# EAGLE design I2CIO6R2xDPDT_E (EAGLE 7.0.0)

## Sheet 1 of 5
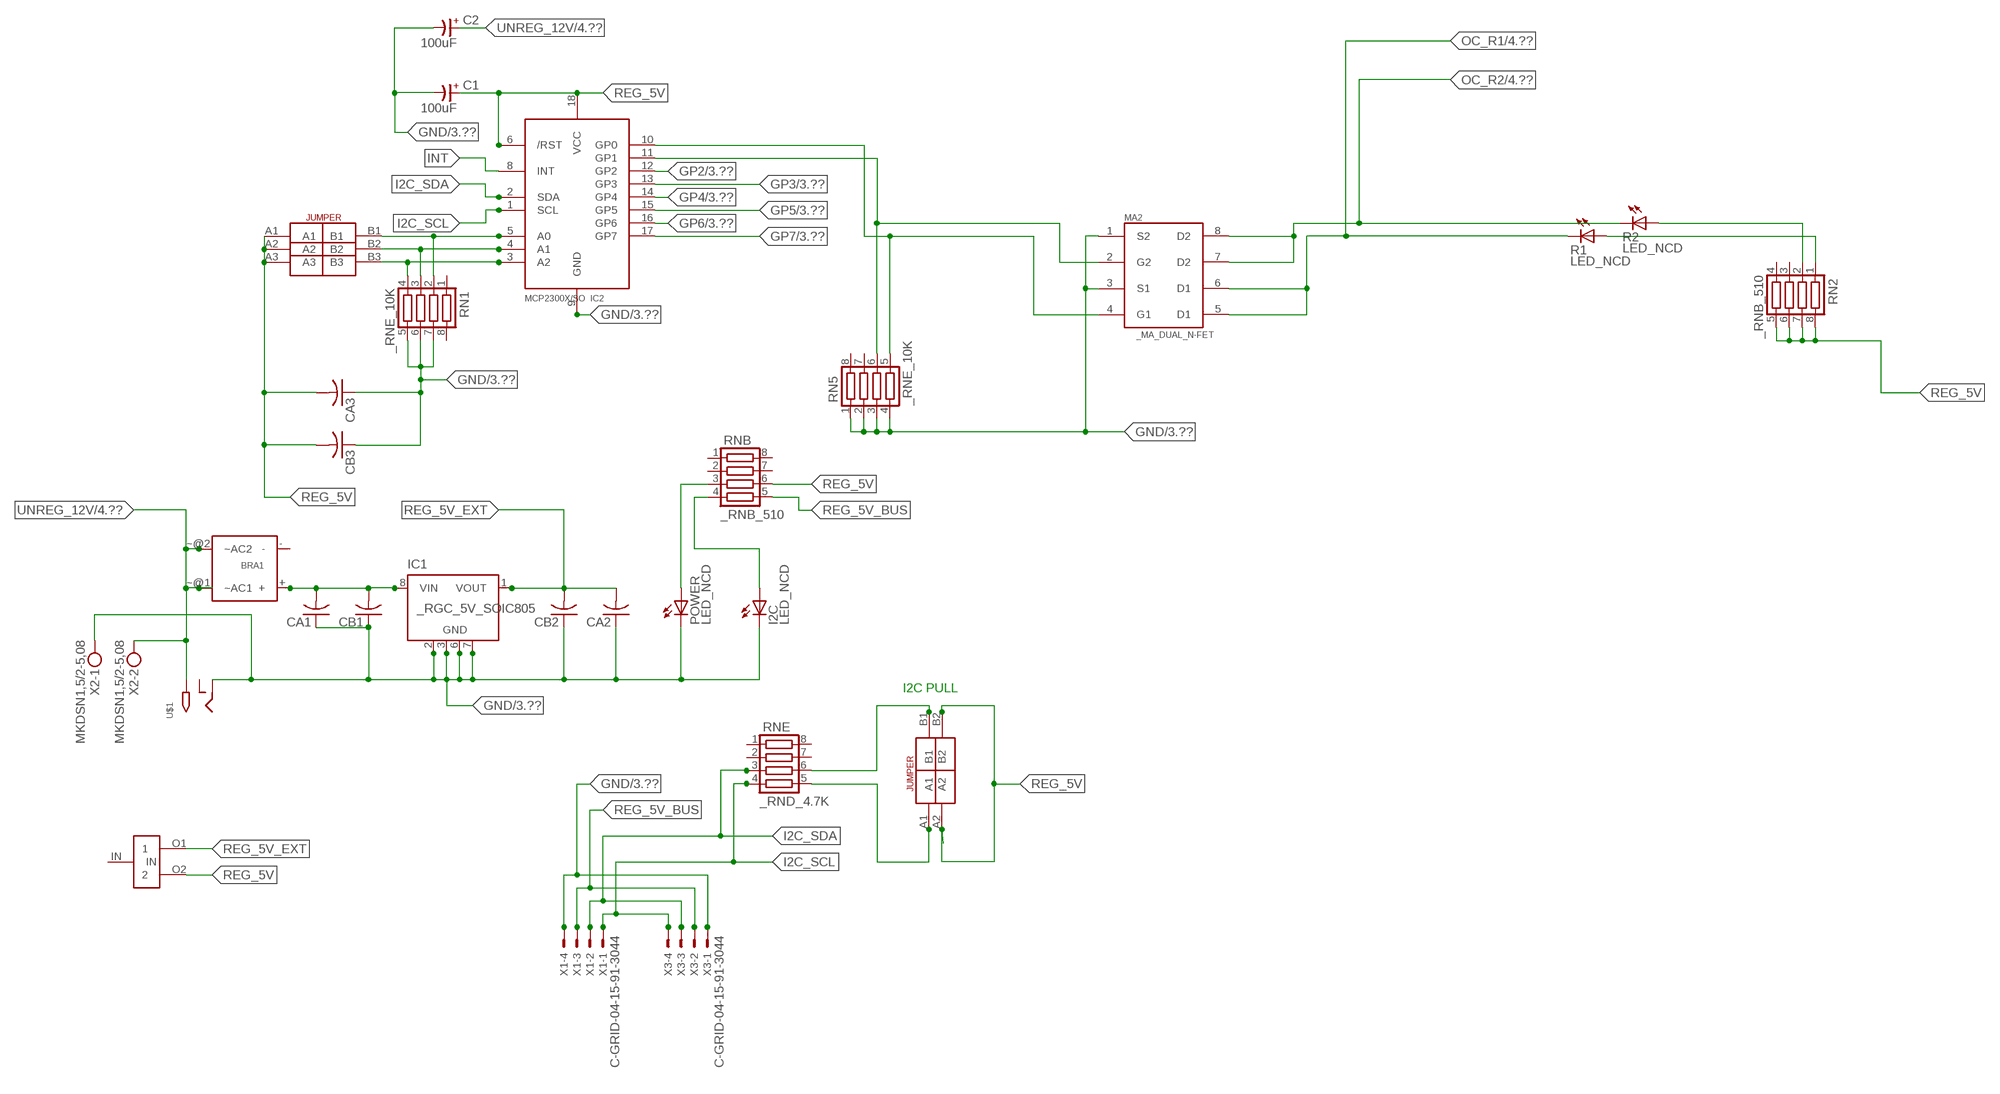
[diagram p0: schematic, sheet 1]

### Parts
BRA1  MB2S_  [MB2S]
C1  100uF  CP-E-025X060  [E-025X060]
C2  100uF  CP-E-025X060  [E-025X060]
CA1  CC1206KRX7R9BB104C1206K  [CC1206KRX7R9BB104]
CA2  CC1206KRX7R9BB104C1206K  [CC1206KRX7R9BB104]
CA3  CC1206KRX7R9BB104C1206K  [CC1206KRX7R9BB104]
CB1  TMK316F106ZL-TC1206K  [TMK316F106ZL-T]
CB2  TMK316F106ZL-TC1206K  [TMK316F106ZL-T]
CB3  TMK316F106ZL-TC1206K  [TMK316F106ZL-T]
I2C  LED_NCD  [CHIPLED_0603]
IC1  _RGC_5V_SOIC805  [_RGC_5V_SOIC8]
IC2  MCP2300X/SO  [SO18W]
MA2  _MA_DUAL_N-FET  [_MA_DUAL_N-FET]
POWER  LED_NCD  [CHIPLED_0603]
R1  LED_NCD  [CHIPLED_0603]
R2  LED_NCD  [CHIPLED_0603]
RN1  _RNE_10K  [RNE]
RN2  _RNB_510  [RNB]
RN5  _RNE_10K  [RNE]
RNB  _RNB_510  [RNB]
RNE  _RND_4.7K  [RND]
U$1  2.1MMJACK  [PJ-102A]
U$3  JUMPER_2X2  [JUMPER_2X2]
U$5  LINK_2  [LINK_2]
U$18  JUMPER_3X2  [JUMPER_3X2]
X1  C-GRID-04-15-91-3044  [15-91-04]
X2  MKDSN1,5/2-5,08  [MKDSN1,5/2-5,08]
X3  C-GRID-04-15-91-3044  [15-91-04]

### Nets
GND: C1.- C2.- CA1.1 CA2.1 CA3.1 CB1.1 CB2.1 CB3.1 I2C.C IC1.2(GND) IC1.3(GND) IC1.6(GND) IC1.7(GND) IC2.9(GND) MA2.1(S2) MA2.3(S1) POWER.C RN1.5 RN1.6 RN1.7 RN5.1 RN5.2 RN5.3 RN5.4 U$1.RING X1.4 X2.1 X3.1 ; also sheet 3
GP2: IC2.12(GP2) ; also sheet 3
GP3: IC2.13(GP3) ; also sheet 3
GP4: IC2.14(GP4) ; also sheet 3
GP5: IC2.15(GP5) ; also sheet 3
GP6: IC2.16(GP6) ; also sheet 3
GP7: IC2.17(GP7) ; also sheet 3
I2C_SCL: IC2.1(SCL) RNE.4 X1.1 X3.4
I2C_SDA: IC2.2(SDA) RNE.3 X1.2 X3.3
INT: IC2.8(INT)
N$1: BRA1.+ CA1.2 CB1.2 IC1.8(VIN)
N$2: POWER.A RNB.3
N$3: I2C.A RNB.4
N$4: RNE.5 U$3.A1
N$5: RNE.6 U$3.B1
N$6: IC2.5(A0) RN1.2 U$18.B1
N$7: IC2.4(A1) RN1.3 U$18.B2
N$8: IC2.3(A2) RN1.4 U$18.B3
N$22: IC2.11(GP1) MA2.2(G2) RN5.6
N$23: IC2.10(GP0) MA2.4(G1) RN5.5
N$31: R2.A RN2.2
N$32: R1.A RN2.1
OC_R1: MA2.5(D1) MA2.6(D1) R1.C ; also sheet 4
OC_R2: MA2.7(D2) MA2.8(D2) R2.C ; also sheet 4
REG_5V: C1.+ CA3.2 CB3.2 IC2.6(/RST) IC2.18(VCC) RN2.5 RN2.6 RN2.7 RN2.8 RNB.6 U$3.A2 U$3.B2 U$5.O2 U$18.A1 U$18.A2 U$18.A3
REG_5V_BUS: RNB.5 X1.3 X3.2
REG_5V_EXT: CA2.2 CB2.2 IC1.1(VOUT) U$5.O1
UNREG_12V: BRA1.~@1(~AC1) BRA1.~@2(~AC2) C2.+ U$1.TIP X2.2 ; also sheet 4
Unconnected: BRA1.- IC1.4(NC) IC1.5(NC) RN1.1 RN1.8 RN2.3 RN2.4 RN5.7 RN5.8 RNB.1 RNB.2 RNB.7 RNB.8 RNE.1 RNE.2 RNE.7 RNE.8 U$1.RING_SW U$5.IN

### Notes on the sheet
- I2C PULL

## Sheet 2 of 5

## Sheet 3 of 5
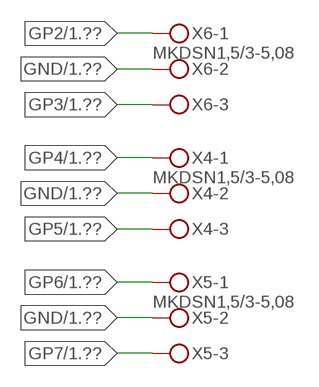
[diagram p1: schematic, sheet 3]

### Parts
X4  MKDSN1,5/3-5,08  [MKDSN1,5/3-5,08]
X5  MKDSN1,5/3-5,08  [MKDSN1,5/3-5,08]
X6  MKDSN1,5/3-5,08  [MKDSN1,5/3-5,08]

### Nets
GND: X4.2 X5.2 X6.2 ; also sheet 1
GP2: X6.1 ; also sheet 1
GP3: X6.3 ; also sheet 1
GP4: X4.1 ; also sheet 1
GP5: X4.3 ; also sheet 1
GP6: X5.1 ; also sheet 1
GP7: X5.3 ; also sheet 1

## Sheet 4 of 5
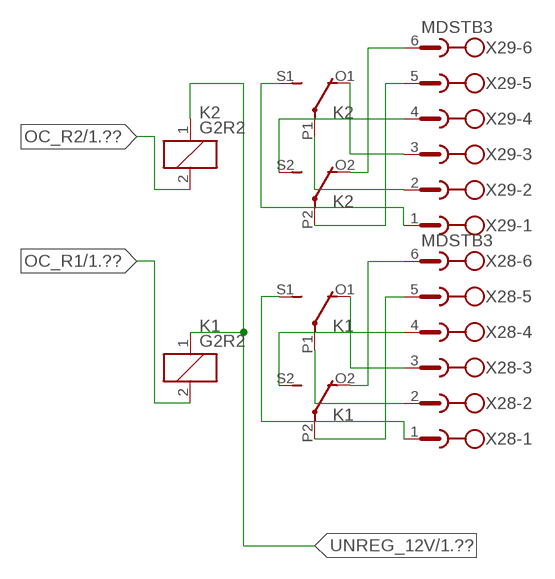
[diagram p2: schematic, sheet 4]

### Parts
K1  G2R2  [G2R2]
K2  G2R2  [G2R2]
X28  MDSTB3  [MDSTB3]
X29  MDSTB3  [MDSTB3]

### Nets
N$203: K1.P2(3:COM) X28.5
N$204: K1.O2(3:NC) X28.6
N$205: K1.S2(3:NO) X28.4
N$206: K1.P1(2:COM) X28.2
N$207: K1.O1(2:NC) X28.3
N$208: K1.S1(2:NO) X28.1
N$209: K2.P2(3:COM) X29.5
N$210: K2.O2(3:NC) X29.6
N$211: K2.S2(3:NO) X29.4
N$212: K2.S1(2:NO) X29.1
N$213: K2.P1(2:COM) X29.2
N$214: K2.O1(2:NC) X29.3
OC_R1: K1.2(1:C2) ; also sheet 1
OC_R2: K2.2(1:C2) ; also sheet 1
UNREG_12V: K1.1(1:C1) K2.1(1:C1) ; also sheet 1

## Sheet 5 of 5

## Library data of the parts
BRA1 = NCD_ULTIMATE_LIBRARY:MB2S: Bridge Rectifier BRA MB2S 200V 500ma Digikey MB2S-TPMSTR-ND/MB2S-TP
C1 C2 = NCD_ULTIMATE_LIBRARY:CP-: Capacitors All Kinds POLARIZED CAP
CA1-CA3 = NCD_ULTIMATE_LIBRARY:CC1206KRX7R9BB104: Capacitor CA .1uF 50V SMT C1206K CC1206KRX7R9BB104
CB1-CB3 = NCD_ULTIMATE_LIBRARY:TMK316F106ZL-T: Capacitor CB 10uF SMT 1206 TMK316F106ZL-T
I2C POWER = NCD_ULTIMATE_bhaskar:LED_NCD
IC1 = NCD_ULTIMATE_LIBRARY:_RGC_5V_SOIC8: Regulator Linear 5V Chip Positive VOLTAGE REGULATOR Digikey 497-7267-2-ND/L78L05CD13TR
IC2 = NCD_ULTIMATE_LIBRARY:MCP2300X: Semiconductor Port Expander I/O 8-Bit I2C MCP23008 Inexpensive i2c i/o expander - 8 general purpose i/o pins with optional pullups
K1 K2 = NCD_ULTIMATE_LIBRARY:G2R2: RELAY 2 x switch, Omron
MA2 = NCD_ULTIMATE_LIBRARY:_MA_DUAL_N-FET: FET Dual N-Channel 8-SOIC NMOSFET Digikey 785-1064-2-ND/AO4842
R1 R2 = NCD_ULTIMATE_LIBRARY:LED_NCD: LED Digikey 754-1132-2-ND/APT2012SRCPRV
RN1 RN5 = NCD_ULTIMATE_LIBRARY:_RNE_10K: Resistor Array RNE SMT 10K x 4 Single Resistor Source: http://www.ctscorp.com/components/Datasheets/CTSChipArrayDs.pdf Digikey 742C083103JPTR-ND/742C083103JP; OC_FARNELL: unknown; OC_NEWARK: unknown
RN2 RNB = NCD_ULTIMATE_LIBRARY:_RNB_510: Resistor Array RNB SMT 510 x 4 Single Resistor Source: http://www.ctscorp.com/components/Datasheets/CTSChipArrayDs.pdf Digikey 742C083511JPTR-ND/ 742C083511JP; OC_FARNELL: unknown; OC_NEWARK: unknown
RNE = NCD_ULTIMATE_LIBRARY:_RND_4.7K: Resistor Array RND SMT 4.7K x 4 Single Resistor Source: http://www.ctscorp.com/components/Datasheets/CTSChipArrayDs.pdf Digikey 742C083472JPTR-ND/742C083472JP; OC_FARNELL: unknown; OC_NEWARK: unknown
U$1 = NCD_ULTIMATE_CONNECTORS:2.1MMJACK: 2.1mm x 5.5mm DC jack with internal switch. Digikey part #PJ-102A, 4UCON part #05537 By microbuilder.eu
U$3 = NCD_ULTIMATE_CONNECTORS:JUMPER_2X2
U$5 = NCD_ULTIMATE_LIBRARY:LINK_2: PAD_top
U$18 = NCD_ULTIMATE_CONNECTORS:JUMPER_3X2
X1 X3 = NCD_ULTIMATE_CONNECTORS:C-GRID-04: CONNECTOR 4-Pos I2C wire to board 2.54 mm (0.100") pitch header Digikey WM1342-ND/0015912045; OC_FARNELL: unknown; OC_NEWARK: unknown
X2 = NCD_ULTIMATE_CONNECTORS:MKDSN1,5/2-5,08: MKDSN 1,5/ 2-5,08 Printklemme
X4-X6 = NCD_ULTIMATE_CONNECTORS:MKDSN1,5/3-5,08: MKDSN 1,5/ 3-5,08 Printklemme Nennstrom: 13,5 A Nennspannung: 250 V Rastermaß: 5,08 mm Polzahl: 3 Anschlussart: Schraubanschluss Montage: Löten Anschlussrichtung Leiter/Platine: 0 ° Artikelnummer: 1729131 Source: http://eshop.phoenixcontact.com .. 1729131.pdf
X28 X29 = NCD_ULTIMATE_LIBRARY:MDSTB3: PHOENIX

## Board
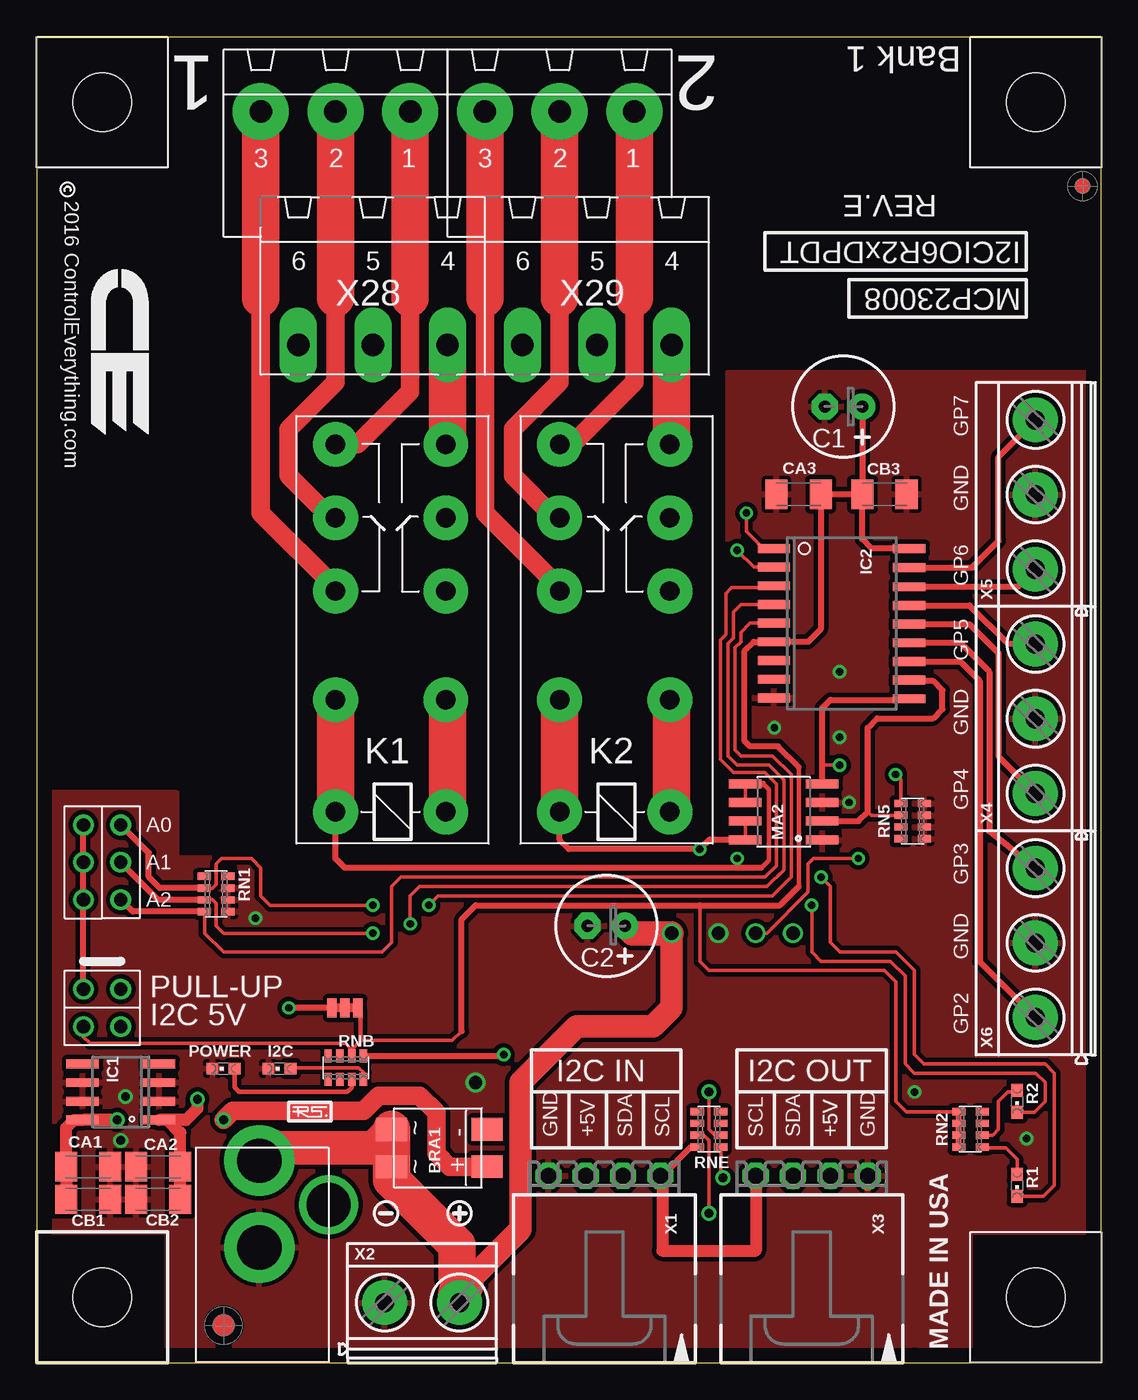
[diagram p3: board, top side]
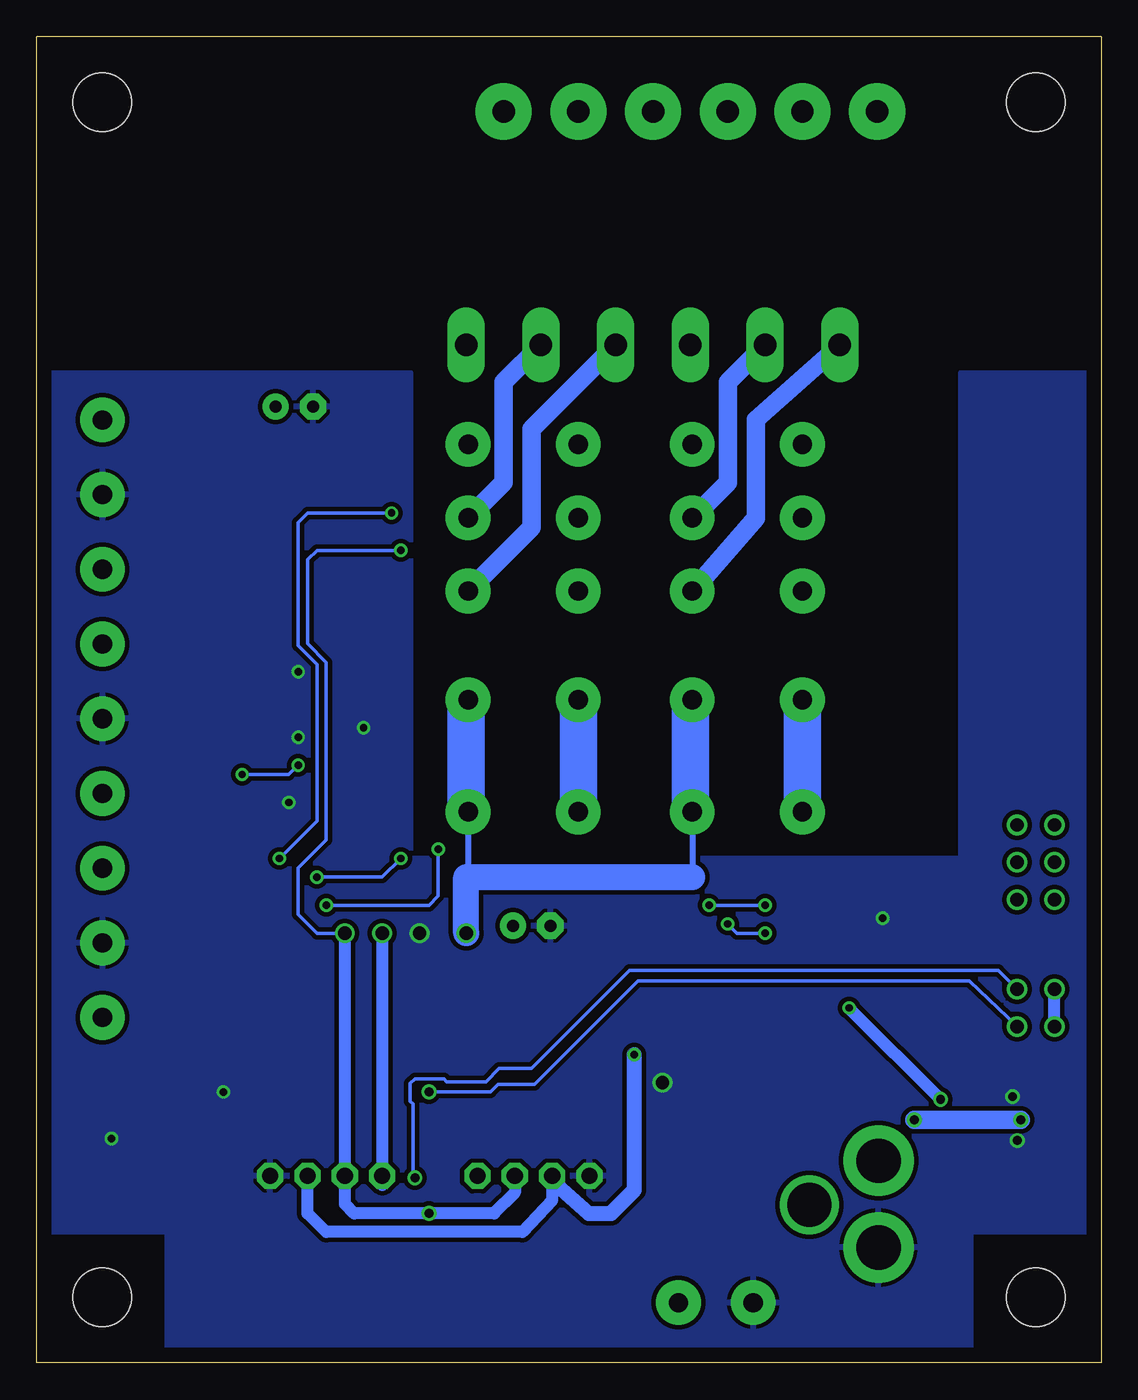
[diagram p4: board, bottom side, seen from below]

Size 72.39 x 90.17 mm. Coordinates in mm from the lower left corner, seen from the top.
Outline: 59.69,0 0,0 0,76.2 0,90.17 72.39,90.17 72.39,0 59.69,0
Outline: 59.69,0 61.58,0
Copper layers (1*16): Top 0.035mm / dielectric 1.5mm / Bottom 0.035mm
Design rules "default": minimum track width 10mil, minimum drill 24mil, track to track 8mil, track to pad 8mil, pad to pad 8mil, via to via 8mil, smd to smd 8mil, copper to edge 40mil, drill to drill 8mil, minimum pad ring 10mil, minimum via ring 8mil, stop-mask expansion 4mil, vias tented up to drill 0mil, thermal gap 10mil
Holes 3.96 mm at 4.45,4.45

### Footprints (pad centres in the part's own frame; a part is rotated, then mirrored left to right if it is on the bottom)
MB2S = smd 1.55 x 2.1: + 0,-6.5; - 2.54,-6.5; ~@1 0,0; ~@2 2.54,0
E-025X060 = drill 0.813 pad 1.778: + -1.27,0 | drill 0.813 pad 1.778 octagon: - 1.27,0
CC1206KRX7R9BB104 = smd 1.5 x 2: 1 -1.5,0; 2 1.5,0
TMK316F106ZL-T = smd 1.5 x 2: 1 -1.5,0; 2 1.5,0
CHIPLED_0603 = smd 0.8 x 0.8: A 0,-0.75; C 0,0.75
_RGC_5V_SOIC8 = smd 0.6 x 2.2: 1 -1.905,-2.6; 2 -0.635,-2.6; 3 0.635,-2.6; 4 1.905,-2.6; 5 1.905,2.6; 6 0.635,2.6; 7 -0.635,2.6; 8 -1.905,2.6
SO18W = smd 0.6 x 2.2: 1 -4.445,-4.6; 2 -3.175,-4.6; 3 -1.905,-4.6; 4 -0.635,-4.6; 5 0.635,-4.6; 6 1.905,-4.6; 7 3.175,-4.6; 8 4.445,-4.6; 9 5.715,-4.6; 10 5.775,4.6; 11 4.505,4.6; 12 3.235,4.6; 13 1.965,4.6; 14 0.695,4.6; 15 -0.575,4.6; 16 -1.845,4.6; 17 -3.145,4.6; 18 -4.445,4.6
G2R2 = drill 1.321 pad 3.048: 1 -2.54,-3.683; 2 -2.54,3.81; 3 5.08,-3.683; 4 5.08,3.81; O1 12.471,3.81; O2 12.471,-3.683; P1 17.45,3.81; P2 17.45,-3.683; S1 22.454,3.81; S2 22.454,-3.683
_MA_DUAL_N-FET = smd 0.61 x 2.21: 1 -1.905,-2.616; 2 -0.635,-2.616; 3 0.635,-2.616; 4 1.905,-2.616; 5 1.905,2.616; 6 0.635,2.616; 7 -0.635,2.616; 8 -1.905,2.616
CHIPLED_0603' = smd 0.8 x 0.876: A 0,-0.75; C 0,0.75
RNE = smd 0.5 x 0.9: 1 -1.2,-0.8; 2 -0.4,-0.8; 3 0.4,-0.8; 4 1.2,-0.8; 5 1.2,0.8; 6 0.4,0.8; 7 -0.4,0.8; 8 -1.2,0.8
RNB = smd 0.5 x 0.9: 1 -1.2,-0.8; 2 -0.4,-0.8; 3 0.4,-0.8; 4 1.2,-0.8; 5 1.2,0.8; 6 0.4,0.8; 7 -0.4,0.8; 8 -1.2,0.8
RND = smd 0.5 x 0.9: 1 -1.2,-0.8; 2 -0.4,-0.8; 3 0.4,-0.8; 4 1.2,-0.8; 5 1.2,0.8; 6 0.4,0.8; 7 -0.4,0.8; 8 -1.2,0.8
PJ-102A = drill 3 pad 4.8: RING 0.1,-3.39; TIP 0.1,-9.29 | drill 3 pad 3.251: RING_SW -4.6,-6.29
JUMPER_2X2 = drill 0.9: A1 0,2.54; A2 0,0; B1 2.54,2.54; B2 2.54,0
PCB_MOUNTING_HOLE = hole 3.962: 4.445,4.445
LINK_2 = smd 1.27 x 0.635: IN 0,0; O1 0,0.889; O2 0,-0.889
JUMPER_3X2 = drill 0.9: A1 0,5.08; A2 0,2.54; A3 0,0; B1 2.54,5.08; B2 2.54,2.54; B3 2.54,0
15-91-04 = drill 1.1 pad 1.778 octagon: 1 -3.81,-7.62; 2 -1.27,-7.62; 3 1.27,-7.62; 4 3.81,-7.62
MKDSN1,5/2-5,08 = drill 1.3 pad 3.048: 1 -2.561,0.025; 2 2.519,0.025
MKDSN1,5/3-5,08 = drill 1.3 pad 3.048: 1 -7.641,0.025; 2 -2.561,0.025; 3 2.519,0.025
MDSTB3 = drill 1.524 pad 3.81: 1 -3.81,-10.795; 2 1.27,-10.795; 3 6.35,-10.795 | drill 1.524 pad 2.54 long: 4 -6.35,5.08; 5 -1.27,5.08; 6 3.81,5.08

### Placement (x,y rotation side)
BRA1  24.13,13.34 90 top
C1  54.86,65.02 180 top
C2  38.73,29.72 180 top
CA1  3.49,13.34 180 top
CA2  8.26,13.34 0 top
CA3  51.82,59.05 0 top
CB1  3.49,11.11 180 top
CB2  8.26,11.11 0 top
CB3  57.66,59.05 180 top
I2C  16.51,20 90 top
IC1  5.71,18.41 90 top
IC2  54.74,50.93 270 top
K1  24.13,40.01 90 top
K2  39.37,40.01 90 top
MA2  50.8,37.47 90 top
POWER  12.7,20 90 top
R1  LED_NCD  [CHIPLED_0603']  66.67,12.06 180 top
R2  LED_NCD  [CHIPLED_0603']  66.67,17.78 180 top
RN1  12.19,31.88 270 top
RN2  63.5,15.88 90 top
RN5  59.56,36.83 90 top
RNB  21.02,20.07 0 top
RNE  45.72,15.88 270 top
U$1  15.24,4.45 180 top
U$3  3.17,25.4 270 top
U$4  PCB_MOUNTING_HOLE  [PCB_MOUNTING_HOLE]  72.39,81.28 90 top
U$5  20.95,24.13 90 top
U$6  PCB_MOUNTING_HOLE  [PCB_MOUNTING_HOLE]  72.39,0 90 top
U$7  PCB_MOUNTING_HOLE  [PCB_MOUNTING_HOLE]  8.89,81.28 90 top
U$10  [VISION_REF15]  12.7,2.54 0 top
U$18  3.17,31.5 0 top
U$19  [VISION_REF10]  71.12,80.01 0 top
U$21  [ICON_USA]  61.98,0.89 90 top
U$22  [ICON_MINUS]  23.75,10.16 180 top
U$24  [ICON_PLUS]  28.77,10.16 90 top
X1  38.61,5.08 180 top
X2  26.23,4.06 0 top
X3  52.7,5.08 180 top
X4  67.94,46.35 90 top
X5  67.94,61.59 90 top
X6  67.94,31.11 90 top
X28  21.59,74.3 180 top
X29  36.83,74.3 180 top

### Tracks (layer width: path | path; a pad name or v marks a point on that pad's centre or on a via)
GND  (via drill 0.5, 0.6, 0.9)
  Top 0.406: 34.8,12.38 X1.4
  Top 0.813: X3.1 56.52,12.06
  other vias: 5.71,15.11 6.03,18.1 46.35,29.21 29.84,19.05 14.86,30.23 54.61,42.55 54.61,46.99 59.69,18.41 67.31,15.24 50.16,43.18 55.24,38.1
  pour Bottom (isolate 0.305): 0.64,8.89 8.89,8.89 8.89,0 63.5,0 63.5,8.89 71.75,8.89 71.75,67.31 46.99,67.31 46.99,34.29 9.53,34.29 9.53,67.31 0.64,67.31
  pour Top (isolate 0.305): 0.64,8.89 8.89,8.89 8.89,0 63.5,0 63.5,8.89 71.75,8.89 71.75,67.31 46.99,67.31 46.99,34.29 9.53,34.29 9.53,38.73 0.64,38.73
GP2
  Top 0.406: IC2.12 62.8,47.69 64.14,46.35 64.14,27.26 X6.1
GP3
  Top 0.406: IC2.13 62.8,48.96 64.77,46.99 64.77,36.15 X6.3
GP4
  Top 0.406: IC2.14 63.43,50.23 65.41,48.26 65.41,41.23 X4.1
GP5
  Top 0.406: IC2.15 63.43,51.5 66.04,48.9 67.9,48.9 X4.3
GP6
  Top 0.406: IC2.16 66.74,52.77 X5.1
GP7
  Top 0.406: IC2.17 63.6,54.07 65.41,55.88 65.41,61.6 X5.3
I2C_SCL  (via drill 0.5, 0.9)
  Top 0.254: IC2.1 49.4,55.37 48.26,56.52 v48.26,57.78 | v55.88,34.29 52.83,34.29 52.45,33.91 52.45,32 49.66,29.21 v48.9,29.21
  Top 0.406: RNE.4 44.51,14.68 42.55,12.7
  Top 0.813: X3.4 48.9,7.62 42.55,7.62 42.55,12.7 X1.1
  Bottom 0.254: v48.26,57.78 53.98,57.78 54.61,57.15 54.61,48.77 53.34,47.5 53.34,36.83 v55.88,34.29
  Bottom 0.813: v48.9,29.21 X3.4 48.9,12.06
I2C_SDA  (via drill 0.5, 0.6, 0.9)
  Top 0.254: RNE.3 45.36,15.47 45.72,15.11 v45.72,10.16 | IC2.2 48.77,54.1 v47.62,55.24
  Top 0.61: X3.3 51.44,12.06 | X1.2 39.88,12.38
  Bottom 0.254: v47.62,55.24 53.34,55.24 53.98,54.61 53.98,48.9 52.7,47.62 52.7,35.56 54.61,33.66 54.61,30.48 53.34,29.21 v51.44,29.21
  Bottom 0.406: 39.88,12.38 X1.2
  Bottom 0.813: 39.88,12.38 39.88,11.56 41.27,10.16 v45.72,10.16 50.8,10.16 51.44,10.79 X3.3 v51.44,29.21
N$1  (via drill 0.6)
  Top 0.813: CB1.2 CA1.2 1.99,15.96 2.54,16.51 IC1.8 v5.46,16.51
  Top 1.27: v12.7,16.51 13.34,17.14 22.23,17.14 23.24,18.16 26.04,18.16 27.18,17.02 27.18,14.22 28.07,13.34 BRA1.+
  Bottom 1.27: v12.7,16.51 v5.46,16.51
N$2
  Top 0.305: RNB.3 21.4,18.95 21.4,18.7 21.12,18.41 13.78,18.41 13.45,18.74 POWER.A
N$3
  Top 0.254: 22.23,18.95 22.23,19.74 21.9,20.07 16.94,20.07
  Top 0.305: RNB.4 22.23,18.95 | 16.94,20.07 I2C.A
N$4  (via drill 0.6)
  Top 0.254: RNE.5 46.52,12.6 v46.67,12.57
  Bottom 0.254: U$3.A1 6.99,26.67 32.07,26.67 38.73,20 40.96,20 41.85,19.11 44.51,19.11 44.7,19.3 46.67,19.3 46.99,18.99 46.99,17.78 46.8,17.59 46.8,12.7 v46.67,12.57
N$5  (via drill 0.6)
  Top 0.254: RNE.6 46.12,15.47 45.72,15.88 v45.72,18.41
  Bottom 0.254: v45.72,18.41 41.53,18.41 41.02,18.92 38.54,18.92 31.5,25.97 8.95,25.97 6.35,23.5 U$3.B1
N$6  (via drill 0.5)
  Top 0.254: v26.67,31.11 27.3,31.75 50.04,31.75 51.31,33.02 51.31,40.01 50.04,41.27 47.88,41.27 47.5,41.66 47.5,48.64 47.88,49.02 47.88,49.66 48.51,50.29 IC2.5 50.01,50.16 | v22.86,31.11 15.88,31.11 15.24,31.75 15.24,33.66 14.61,34.29 12.57,34.29 12.19,33.91 12.19,32.51 11.94,32.26 11.41,32.26 RN1.2
  Top 0.406: RN1.2 8.36,32.28 7.62,33.02 7.62,34.67 U$18.B1
  Bottom 0.254: v26.67,31.11 v22.86,31.11
N$7  (via drill 0.5)
  Top 0.254: v25.4,29.84 25.4,31.75 26.04,32.38 49.66,32.38 50.8,33.53 50.8,39.62 49.78,40.64 47.62,40.64 46.99,41.27 46.99,48.9 47.37,49.28 47.37,51.05 47.88,51.56 IC2.4 50.01,51.44 | v22.86,29.21 12.7,29.21 12.19,29.72 12.19,31.24 11.94,31.5 11.41,31.5 RN1.3
  Top 0.406: RN1.3 8.27,31.48 U$18.B2
  Bottom 0.254: v25.4,29.84 24.77,29.21 v22.86,29.21
N$8
  Top 0.254: RN1.4 11.43,30.64 11.43,29.21 12.7,27.94 23.5,27.94 24.13,28.57 24.13,32.38 24.77,33.02 49.53,33.02 50.29,33.78 50.29,39.37 49.53,40.13 47.37,40.13 46.48,41.02 46.48,49.15 46.86,49.53 46.86,52.32 47.24,52.7 50.01,52.7 IC2.3
  Top 0.406: RN1.4 6.53,30.68 U$18.B3
N$22
  Top 0.254: RN5.6 56.75,37.23 56.52,37.47
  Top 0.406: MA2.2 55.88,36.83 56.52,37.47 56.52,43.18 57.15,43.81 60.96,43.81 61.59,44.45 61.59,45.72 60.96,46.35 59.4,46.35 IC2.11
N$23  (via drill 0.5)
  Top 0.254: RN5.5 58.76,39.66 v58.42,40.01 | v54.61,40.64 53.42,40.64
  Top 0.406: MA2.4 53.42,40.64 53.42,44.53 53.98,45.09 59.27,45.09 IC2.10
  Bottom 0.254: v58.42,40.01 55.24,40.01 v54.61,40.64
N$31
  Top 0.254: RN2.2 65,15.47 65.41,15.88 65.41,17.78 66.04,18.41 66.56,18.41 R2.A
N$32
  Top 0.254: R1.A 66.67,13.84 65.91,14.61 64.37,14.61 RN2.1
N$203
  Bottom 1.27: X28.5 25.4,66.67 25.4,59.87 K1.P2
N$204
  Bottom 1.27: X28.6 23.5,64.14 23.5,57.43 K1.O2
N$205
  Top 2.54: X28.4 27.94,62.59 K1.S2
N$206
  Top 1.27: K1.P1 20.02,57.45 17.14,60.33 17.14,63.5 20.32,66.67 20.32,72.39
  Top 2.54: X28.2 20.32,72.39
N$207
  Top 1.27: K1.O1 20.32,52.7 15.24,57.78 15.24,72.39
  Top 2.54: X28.3 15.24,72.39
N$208
  Top 1.27: 25.4,72.39 25.4,66.04 21.82,62.46 K1.S1
  Top 2.54: X28.1 25.4,72.39
N$209
  Bottom 1.27: X29.5 40.64,66.67 40.64,59.87 K2.P2
N$210
  Bottom 1.27: X29.6 38.73,63.5 38.73,56.79 K2.O2
N$211
  Top 2.54: X29.4 43.18,62.59 K2.S2
N$212
  Top 1.27: 40.64,72.39 40.64,66.67 36.42,62.46 K2.S1
  Top 2.54: X29.1 40.64,72.39
N$213
  Top 1.27: K2.P1 35.26,57.45 32.38,60.33 32.38,63.5 35.56,66.67 35.56,72.39
  Top 2.54: X29.2 35.56,72.39
N$214
  Top 1.27: K2.O1 35.56,52.7 30.48,57.78 30.48,72.39
  Top 2.54: X29.3 30.48,72.39
OC_R1  (via drill 0.5)
  Top 0.254: MA2.5 MA2.6 | R1.C 68.47,11.31 69.22,12.06 69.22,19.68 68.58,20.32 60.33,20.32 59.69,20.95 59.69,26.67 58.42,27.94 54.61,27.94 53.98,28.57 53.98,32.38 v53.34,33.02 | v47.62,34.29 47.62,33.66
  Top 0.305: 49.4,39.37 49.78,38.99 49.78,34.16 49.28,33.66
  Top 0.406: MA2.5 49.4,39.37 | 49.28,33.66 47.62,33.66 20.95,33.66 20.32,34.29 K1.2
  Bottom 0.254: v53.34,33.02 48.9,33.02 v47.62,34.29
OC_R2  (via drill 0.5)
  Top 0.254: MA2.7 MA2.8 | R2.C 67.83,17.03 68.58,17.78 68.58,19.05 67.94,19.68 59.69,19.68 59.05,20.32 59.05,26.29 58.04,27.3 53.34,27.3 52.7,27.94 v52.7,31.11
  Top 0.406: MA2.8 45.72,35.56 v45.09,34.92 36.2,34.92 35.56,35.56 K2.2
  Bottom 0.254: v52.7,31.11 45.72,31.11 45.09,31.75 v45.09,34.92
REG_5V
  Top 0.254: RNB.6 21.42,21.29 | 21.42,21.29 22.04,21.91 28.26,21.91 28.89,22.54 | 21.42,21.29 20.99,21.72 3.62,21.72 3.17,22.16 U$3.B2 | RN2.5 59.12,17.07 58.42,17.78 58.42,25.91 57.66,26.67 45.72,26.67 45.09,27.3 45.09,31.11
  Top 0.305: 51.82,32.38 51.82,40.51 | 22.04,21.91 22.04,23.94 U$5.O2
  Top 0.406: U$18.A1 U$18.A2 U$18.A3 U$3.A2 | RN2.8 RN2.7 RN2.6 RN2.5 | 28.89,22.54 28.89,30.16 29.84,31.11 45.09,31.11 50.55,31.11 51.82,32.38 | 51.82,40.51 50.42,41.91 48.51,41.91 48.13,42.29 48.13,48.39 48.77,49.02 IC2.6 52.45,49.02 53.32,49.89 CA3.2 CB3.2 56.13,59.03 | IC2.18 56.77,55.37 56.13,56.01 56.13,59.03 | C1.+ 56.13,59.03
  Bottom 0.813: U$3.B2 U$3.A2
REG_5V_BUS  (via drill 0.5)
  Top 0.406: RNB.5 31.66,20.87 v31.75,20.95
  Top 0.61: X1.3 37.34,12.38 | X3.2 53.98,12.06
  Bottom 0.406: 37.34,12.38 X1.3 | 53.98,12.06 X3.2
  Bottom 0.813: 37.34,12.38 37.34,11.05 39.37,8.89 52.7,8.89 53.98,10.16 53.98,12.06
  Bottom 1.016: 37.34,12.38 34.86,10.16 33.34,10.16 31.75,11.75 v31.75,20.95
REG_5V_EXT  (via drill 0.5, 0.6)
  Top 0.406: U$5.O1 v17.14,24.13
  Top 0.813: CB2.2 CA2.2 9.76,15.64 8.89,16.51 | 8.89,16.51 IC1.1 | v10.92,17.91 10.92,17.27 10.16,16.51 8.89,16.51
  Bottom 0.813: v17.14,24.13 v10.92,17.91
UNREG_12V  (via drill 0.9)
  Top 1.524: v43.18,29.21 43.18,24.13 41.91,22.86 36.7,22.86 32.89,19.05 32.89,9.08 29.11,5.3 28.57,4.76
  Top 1.676: v43.18,29.21 40.51,29.21 C2.+
  Top 2.286: BRA1.~@2 22.86,14.61 16.01,14.61
  Top 2.54: 16.01,14.61 U$1.TIP | X2.2 28.55,4.45 28.57,4.76 | BRA1.~@2 BRA1.~@1 24.13,12.45 28.57,8 28.57,5.84 29.11,5.3
  Bottom 0.406: K2.1 43.05,33.15 43.18,33.02 | K1.1 27.81,33.15 27.94,33.02
  Bottom 1.778: v43.18,29.21 43.18,33.02 27.94,33.02 27.81,33.02

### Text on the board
tNames: Bank 1 | 1 | 2 | 2016 ControlEverything.com | REV.E | I2CIO6R2xDPDT | MCP23008 | GP7 | GND | GP6 | GP5 | GND | GP4 | A0 | A1 | GP3 | A2 | GND | PULL-UP | I2C 5V | GP2 | I2C IN | I2C OUT | GND | +5V | SDA | SCL | SCL | SDA | +5V | +5V | GND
